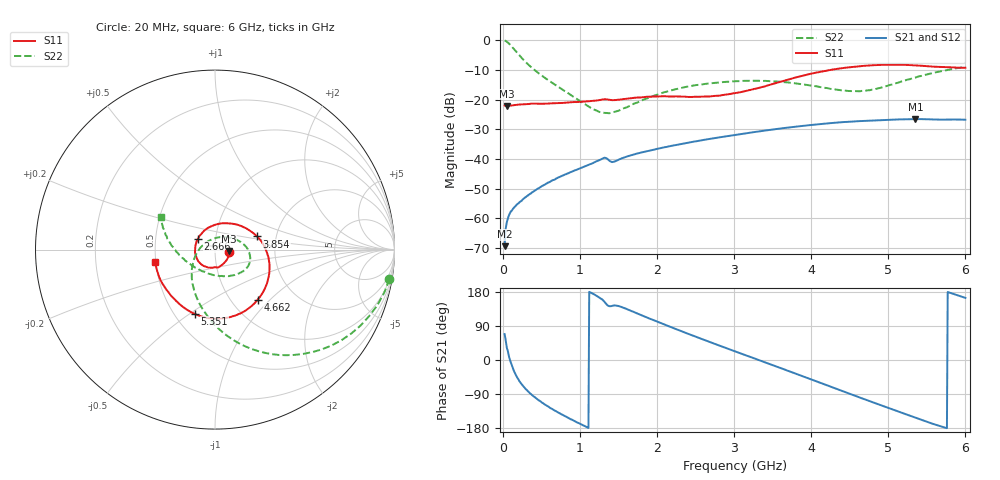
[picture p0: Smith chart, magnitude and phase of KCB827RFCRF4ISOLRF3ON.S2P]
!Agilent Technologies,E5071B,JP1KK00126,A.08.11
!Date: Tue May 06 07:11:58 2014
!Data & Calibration Information:
!Freq	S11:SOLT2(ON)	S21:SOLT2(ON)	S12:SOLT2(ON)	S22:SOLT2(ON)
# Hz S dB R 50
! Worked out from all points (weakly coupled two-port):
!   600 points, 20 MHz to 6 GHz, reference 50 ohm
!   highest |S21| = -26.57 dB at 5.351 GHz (marker M1); lowest = -69.3 dB at 20 MHz (marker M2)
!   lowest |S11| = -22.2 dB at 49.95 MHz (marker M3), VSWR 1.17, Z = 58.4 - j0.885 ohm
!   |S11| at or under -10 dB: start of sweep to 4.257 GHz
!   |S22| runs from -24.6 to -0.1 dB; largest |S21 - S12| = 0.0003
!   S11 on the Smith chart (normalised r, x): 20 MHz: 1.17, -0.04; 2.666 GHz: 0.82, +0.10; 3.854 GHz: 1.59, +0.25; 4.662 GHz: 1.31, -0.85; 5.351 GHz: 0.63, -0.53; 6 GHz: 0.49, -0.08
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2e7  -21.98 -11.3  -69.34 68.4  -67.99 66.8  -0.12 -9.6
4.994992e7  -22.15 -5.5  -61.10 31.1  -61.05 30.5  -0.58 -23.3
7.989983e7  -22.09 -5.3  -58.73 6.6  -58.72 8.9  -1.24 -35.7
1.397997e8  -21.90 -7.2  -56.44 -28.3  -56.52 -29.3  -2.99 -56.1
2.196661e8  -21.66 -11.0  -54.41 -58.0  -54.50 -58.1  -5.38 -75.7
3.194992e8  -21.55 -18.2  -52.38 -82.1  -52.33 -81.9  -8.05 -93.2
5.590985e8  -21.40 -33.0  -48.31 -119.4  -48.37 -119.8  -13.00 -124.2
1.018331e9  -20.73 -59.8  -42.97 -170.1  -42.95 -170.4  -20.90 -178.9
1.297863e9  -19.97 -78.6  -39.76 157.6  -39.80 157.6  -24.46 126.4
1.37773e9  -20.09 -86.5  -40.49 141.9  -40.52 141.9  -24.61 109.8
1.437629e9  -20.19 -89.5  -40.95 144.0  -40.97 143.9  -24.19 97.5
2.016661e9  -18.98 -138.7  -36.51 100.0  -36.52 99.8  -18.22 28.8
2.665576e9  -18.97 148.2  -33.32 48.8  -33.33 48.8  -14.59 -1.4
3.014992e9  -17.83 104.8  -31.89 22.4  -31.87 22.4  -13.85 -14.6
3.474224e9  -14.97 52.8  -30.17 -11.8  -30.17 -12.0  -13.82 -31.3
3.853589e9  -12.18 17.4  -28.98 -40.3  -28.97 -40.4  -14.76 -48.6
4.013322e9  -11.21 4.0  -28.53 -52.3  -28.53 -52.5  -15.38 -58.4
4.342771e9  -9.65 -23.4  -27.74 -77.4  -27.74 -77.5  -16.70 -84.9
4.662237e9  -8.71 -49.6  -27.22 -101.5  -27.21 -101.7  -17.07 -120.2
5.011653e9  -8.28 -78.1  -26.81 -127.2  -26.80 -127.5  -15.17 -158.4
5.351085e9  -8.49 -107.4  -26.57 -152.2  -26.58 -152.4  -12.61 176.7
6e9  -9.32 -168.3  -26.80 163.9  -26.80 163.8  -9.03 148.8
